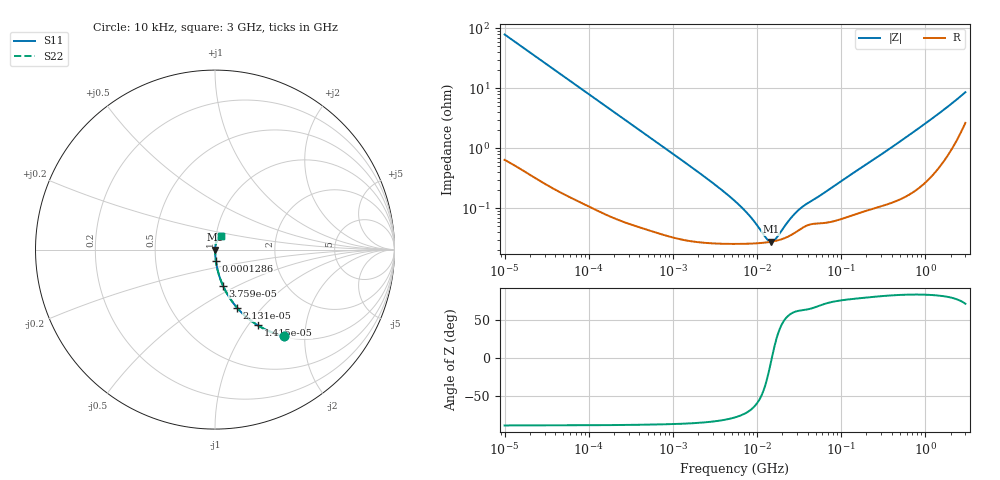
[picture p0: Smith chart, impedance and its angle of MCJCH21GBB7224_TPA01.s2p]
! MCJCH21GBB7224_TPA01  S-PARAMETER MODEL  ( Standard Model )
! Model Generated by TAIYO YUDEN Corporation (http://www.ty-top.com)
! Version 1.0
! TAIYO YUDEN Control No. 220601
! Copyright(c) 2015 TAIYO YUDEN CO.,LTD. All Rights Reserved.
! Product Description (link to TY-COMPAS)
! https://ds.yuden.co.jp/TYCOMPAS/or/detail?pn=MCJCH21GBB7224KTPA01&u=M
! Products Name : Multilayer Ceramic Capacitors
! Characteristics :
!  Capacitance : 0.22 [uF] , Rated Voltage : 100 [V] , TCC : X7R
!  Case Size : 2.0 x 1.25 / 0.079 x 0.049 [mm/inch] , Thickness : 1.25 / 0.049 [mm/inch]
!  (Conditions: Temperature = 25 [degC] , DC Bias Voltage = 0 [V])
! External Node Assignments :
!  1  o---| |---o  2
! GND o---------o GND
! Frequency Range : 10kHz  -  3GHz  [ 401 STEP ]
# MHZ S RI R 50
! Freq[MHz].  S11 Real  S11 Imag  S21 Real  S21 Imag  S12 Real  S12 Imag  S22 Real  S22 Imag
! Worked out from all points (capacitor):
!   401 points, 10 kHz to 3 GHz, reference 50 ohm
!   read as one part in series: C = 202 nF near 10.65 kHz
!   lowest |Z| = 27.9 mohm at 14.56 MHz (marker M1)
!   series resonance near 15.01 MHz, so ESL is about 560 pH
!   S11 on the Smith chart (normalised r, x): 10 kHz: 1.01, -1.57; 14.15 kHz: 1.01, -1.11; 21.31 kHz: 1.01, -0.74; 37.59 kHz: 1.00, -0.42; 128.6 kHz: 1.00, -0.12; 3 GHz: 1.05, +0.16
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0.01  0.3834 -0.4822  0.6166 0.4822  0.6166 0.4822  0.3834 -0.4822
0.014146  0.2391 -0.4222  0.7609 0.4222  0.7609 0.4222  0.2391 -0.4222
0.021312  0.1232 -0.3241  0.8768 0.3241  0.8768 0.3241  0.1232 -0.3241
0.037592  0.0445 -0.2011  0.9555 0.2011  0.9555 0.2011  0.0445 -0.2011
0.082683  0.0104 -0.0952  0.9896 0.0952  0.9896 0.0952  0.0104 -0.0952
0.128563  0.00474 -0.0618  0.9953 0.0618  0.9953 0.0618  0.00474 -0.0618
0.265492  0.0015 -0.0302  0.9985 0.0302  0.9985 0.0302  0.0015 -0.0302
0.683653  0.00052 -0.0118  0.9995 0.0118  0.9995 0.0118  0.00052 -0.0118
2.652321  0.000272 -0.00298  0.9997 0.00298  0.9997 0.00298  0.000272 -0.00298
5.477226  0.000257 -0.00129  0.9997 0.00129  0.9997 0.00129  0.000257 -0.00129
8.516475  0.000259 -0.000651  0.9997 0.000651  0.9997 0.000651  0.000259 -0.000651
12.83117  0.00027 -0.000172  0.9997 0.000172  0.9997 0.000172  0.00027 -0.000172
14.55585  0.000277 -3.33e-05  0.9997 3.33e-05  0.9997 3.33e-05  0.000277 -3.33e-05
15.50326  0.000281 3.56e-05  0.9997 -3.56e-05  0.9997 -3.56e-05  0.000281 3.56e-05
17.04125  0.000289 0.000139  0.9997 -0.000139  0.9997 -0.000139  0.000289 0.000139
23.35767  0.000337 0.000496  0.9997 -0.000496  0.9997 -0.000496  0.000337 0.000496
29.12589  0.000404 0.000754  0.9996 -0.000754  0.9996 -0.000754  0.000404 0.000754
35.19136  0.00048 0.000964  0.9995 -0.000964  0.9995 -0.000964  0.00048 0.000964
45.28751  0.000549 0.00123  0.9995 -0.00123  0.9995 -0.00123  0.000549 0.00123
374.4521  0.00129 0.00968  0.9987 -0.00968  0.9987 -0.00968  0.00129 0.00968
1202.347  0.0044 0.0308  0.9956 -0.0308  0.9956 -0.0308  0.0044 0.0308
3000  0.032 0.077  0.968 -0.077  0.968 -0.077  0.032 0.077
